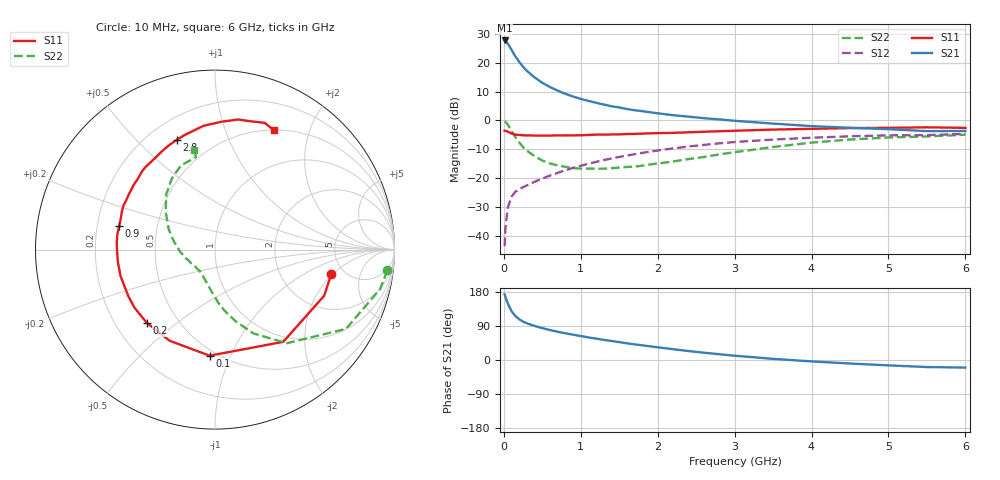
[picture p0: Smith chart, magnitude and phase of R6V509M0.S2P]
! SIEMENS Small Signal Semiconductors
! BFR193
! Si NPN RF Bipolar Junction Transistor in SOT23
! VCE = 0.5 V  IC = 9 mA
! Common Emitter S-Parameters:  May  1996
# GHz  S  MA  R  50
!  f  S11  S21  S12  S22
! GHz  MAG  ANG  MAG  ANG  MAG  ANG  MAG  ANG
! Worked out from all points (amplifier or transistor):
!   36 points, 10 MHz to 6 GHz, reference 50 ohm
!   highest |S21| = 27.7 dB at 10 MHz (marker M1)
!   |S21| within 3 dB of that: start of sweep to 94.66 MHz
!   unconditionally stable (mu >= 1): 679 MHz to 2.519 GHz
!   at 250 MHz: K = 0.63, MSG = 20.9 dB, |S12| = -23.1 dB
!   at 1.4 GHz: K = 1.07, MAG = 7.5 dB, |S12| = -13.2 dB
!   at 6 GHz: K = 1.00, MSG = 0.5 dB, |S12| = -4.7 dB
!   S11 on the Smith chart (normalised r, x): 10 MHz: 3.94, -1.92; 100 MHz: 0.46, -0.84; 200 MHz: 0.33, -0.39; 900 MHz: 0.29, +0.11; 2.8 GHz: 0.31, +0.67; 6 GHz: 0.51, +1.49
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0.01  0.6622 -11.9  24.29 173.5  0.0066 84.7  0.9669 -6.9
0.02  0.6603 -22.9  23.75 166.9  0.0134 77.2  0.9462 -13.4
0.05  0.6391 -53.5  21.56 149.7  0.0303 67.1  0.8531 -31.2
0.1  0.5919 -92.9  16.73 128.9  0.0479 54.6  0.6572 -52.5
0.15  0.5671 -116.5  12.83 116.0  0.0579 48.7  0.513 -65.5
0.2  0.5577 -132.9  10.32 107.5  0.0637 47.1  0.4137 -74.1
0.25  0.5532 -144.2  8.491 101.2  0.0696 47.0  0.3439 -81.2
0.3  0.5482 -151.9  7.2 96.7  0.0746 47.9  0.2984 -86.2
0.4  0.5464 -164.2  5.556 89.9  0.0863 49.8  0.2396 -93.9
0.5  0.5454 -172.0  4.484 84.1  0.0979 52.1  0.2012 -101.1
0.6  0.5458 -178.8  3.78 79.0  0.1104 53.6  0.1789 -107.5
0.7  0.549 175.6  3.275 74.5  0.1232 54.7  0.1656 -112.6
0.9  0.5501 166.2  2.591 66.8  0.1501 55.4  0.1488 -122.3
1.1  0.5599 158.2  2.176 59.6  0.1773 55.2  0.1459 -132.1
1.3  0.5661 150.9  1.881 53.1  0.2052 53.9  0.1453 -141.5
1.6  0.5795 141.2  1.572 44.1  0.2456 51.2  0.156 -153.4
2.2  0.6073 124.4  1.231 28.5  0.3266 43.8  0.1937 -176.0
2.8  0.6483 109.0  1.04 15.2  0.4 34.9  0.2574 161.9
3.5  0.6928 95.2  0.88 3.0  0.4653 23.6  0.3459 142.6
4.5  0.7358 80.0  0.744 -9.3  0.5298 9.4  0.4656 120.9
5.5  0.7584 68.6  0.651 -18.6  0.5537 -3.9  0.5267 101.6
6  0.7414 63.6  0.656 -20.0  0.5847 -8.0  0.564 101.7
